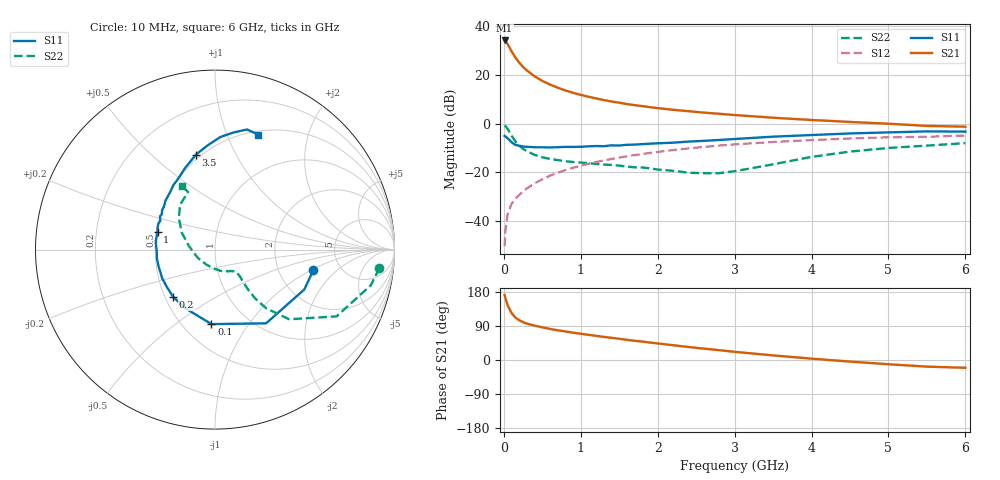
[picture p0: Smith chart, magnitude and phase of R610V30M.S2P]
! SIEMENS Small Signal Semiconductors
! BFR193
! Si NPN RF Bipolar Junction Transistor in SOT23
! VCE = 10 V  IC = 30 mA
! Common Emitter S-Parameters:  May  1996
# GHz  S  MA  R  50
!  f  S11  S21  S12  S22
! GHz  MAG  ANG  MAG  ANG  MAG  ANG  MAG  ANG
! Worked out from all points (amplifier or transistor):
!   36 points, 10 MHz to 6 GHz, reference 50 ohm
!   highest |S21| = 34.0 dB at 10 MHz (marker M1)
!   |S21| within 3 dB of that: start of sweep to 75.32 MHz
!   unconditionally stable (mu >= 1): 529.9 MHz to 2.174 GHz
!   at 250 MHz: K = 0.87, MSG = 25.4 dB, |S12| = -27.7 dB
!   at 1.4 GHz: K = 1.02, MAG = 10.8 dB, |S12| = -14.5 dB
!   at 6 GHz: K = 0.94, MSG = 1.8 dB, |S12| = -4.9 dB
!   S11 on the Smith chart (normalised r, x): 10 MHz: 3.15, -1.06; 100 MHz: 0.68, -0.69; 200 MHz: 0.55, -0.33; 1 GHz: 0.51, +0.11; 3.5 GHz: 0.47, +0.70; 6 GHz: 0.54, +1.30
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0.01  0.5599 -11.9  50.25 171.3  0.0031 71.8  0.9217 -6.4
0.02  0.5448 -24.1  48.83 163.6  0.0062 76.6  0.8906 -12.9
0.05  0.4997 -55.3  42.07 144.4  0.0141 67.9  0.7724 -28.8
0.1  0.4156 -92.7  30.21 124.0  0.0227 63.8  0.567 -43.2
0.15  0.3667 -116.4  22.48 112.0  0.0289 63.2  0.4338 -48.9
0.2  0.3518 -131.6  17.66 105.0  0.0347 65.0  0.3563 -50.5
0.25  0.3392 -142.4  14.4 99.9  0.0411 66.0  0.3043 -50.6
0.3  0.335 -151.4  12.19 96.2  0.0472 68.1  0.2709 -50.0
0.4  0.3277 -163.7  9.3 90.7  0.0599 69.3  0.2295 -48.5
0.5  0.3275 -171.2  7.482 86.1  0.0724 69.9  0.2041 -47.1
0.6  0.3247 -177.9  6.295 82.1  0.0858 70.1  0.1895 -46.7
0.7  0.3287 176.8  5.433 78.4  0.0985 69.9  0.179 -46.9
0.8  0.3336 171.6  4.769 75.3  0.1115 69.0  0.1699 -47.4
1  0.3351 162.9  3.864 69.3  0.1375 67.5  0.1591 -49.1
1.1  0.3426 159.4  3.545 66.4  0.1507 66.3  0.1551 -51.4
1.6  0.3681 143.2  2.508 53.2  0.214 60.2  0.1317 -64.4
2.2  0.4066 127.8  1.916 39.0  0.2871 51.9  0.108 -91.2
2.8  0.4625 113.8  1.587 25.9  0.3548 43.2  0.0967 -138.0
3.5  0.5399 101.3  1.318 12.1  0.4202 32.4  0.1467 172.3
4.5  0.6285 87.2  1.081 -4.2  0.4958 18.7  0.2672 138.9
5.5  0.6927 75.1  0.896 -17.5  0.537 4.9  0.354 115.1
6  0.6847 69.3  0.864 -20.5  0.5711 1.1  0.3984 117.4
